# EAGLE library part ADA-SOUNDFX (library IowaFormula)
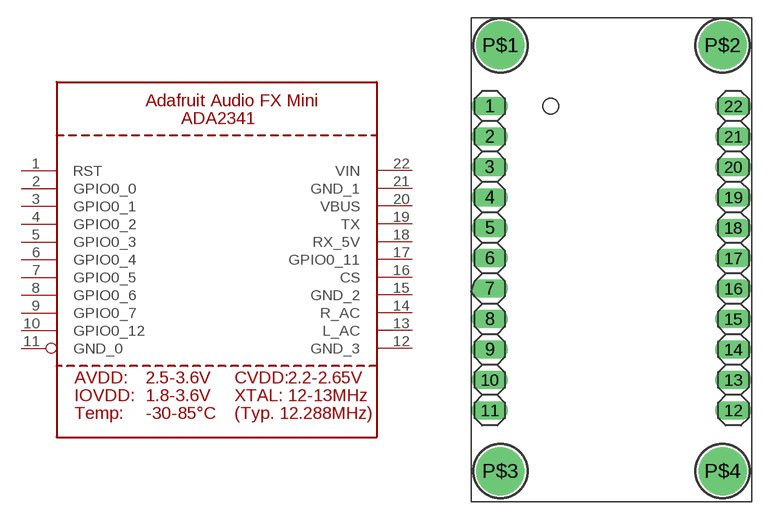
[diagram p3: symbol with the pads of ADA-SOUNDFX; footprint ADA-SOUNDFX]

Designator prefix -

## ADA-SOUNDFX  [ADA-SOUNDFX]
1  RST
2  GPIO0_0
3  GPIO0_1
4  GPIO0_2
5  GPIO0_3
6  GPIO0_4
7  GPIO0_5
8  GPIO0_6
9  GPIO0_7
10  GPIO0_12
11  GND_0  sup
12  GND_3  sup
13  L_AC
14  R_AC
15  GND_2
16  CS
17  GPIO0_11
18  RX_5V
19  TX
20  VBUS
21  GND_1  sup
22  VIN  sup

## Footprint ADA-SOUNDFX (pad centres in mm)
drill 1.016 long: 1 0,25.4; 2 0,22.86; 3 0,20.32; 4 0,17.78; 5 0,15.24; 6 0,12.7; 7 0,10.16; 8 0,7.62; 9 0,5.08; 10 0,2.54; 11 0,0; 12 20.32,0; 13 20.32,2.54; 14 20.32,5.08; 15 20.32,7.62; 16 20.32,10.16; 17 20.32,12.7; 18 20.32,15.24; 19 20.32,17.78; 20 20.32,20.32; 21 20.32,22.86; 22 20.32,25.4
drill 2.5 pad 4: P$1 0.889,30.48; P$2 19.431,30.48; P$3 0.889,-5.08; P$4 19.431,-5.08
